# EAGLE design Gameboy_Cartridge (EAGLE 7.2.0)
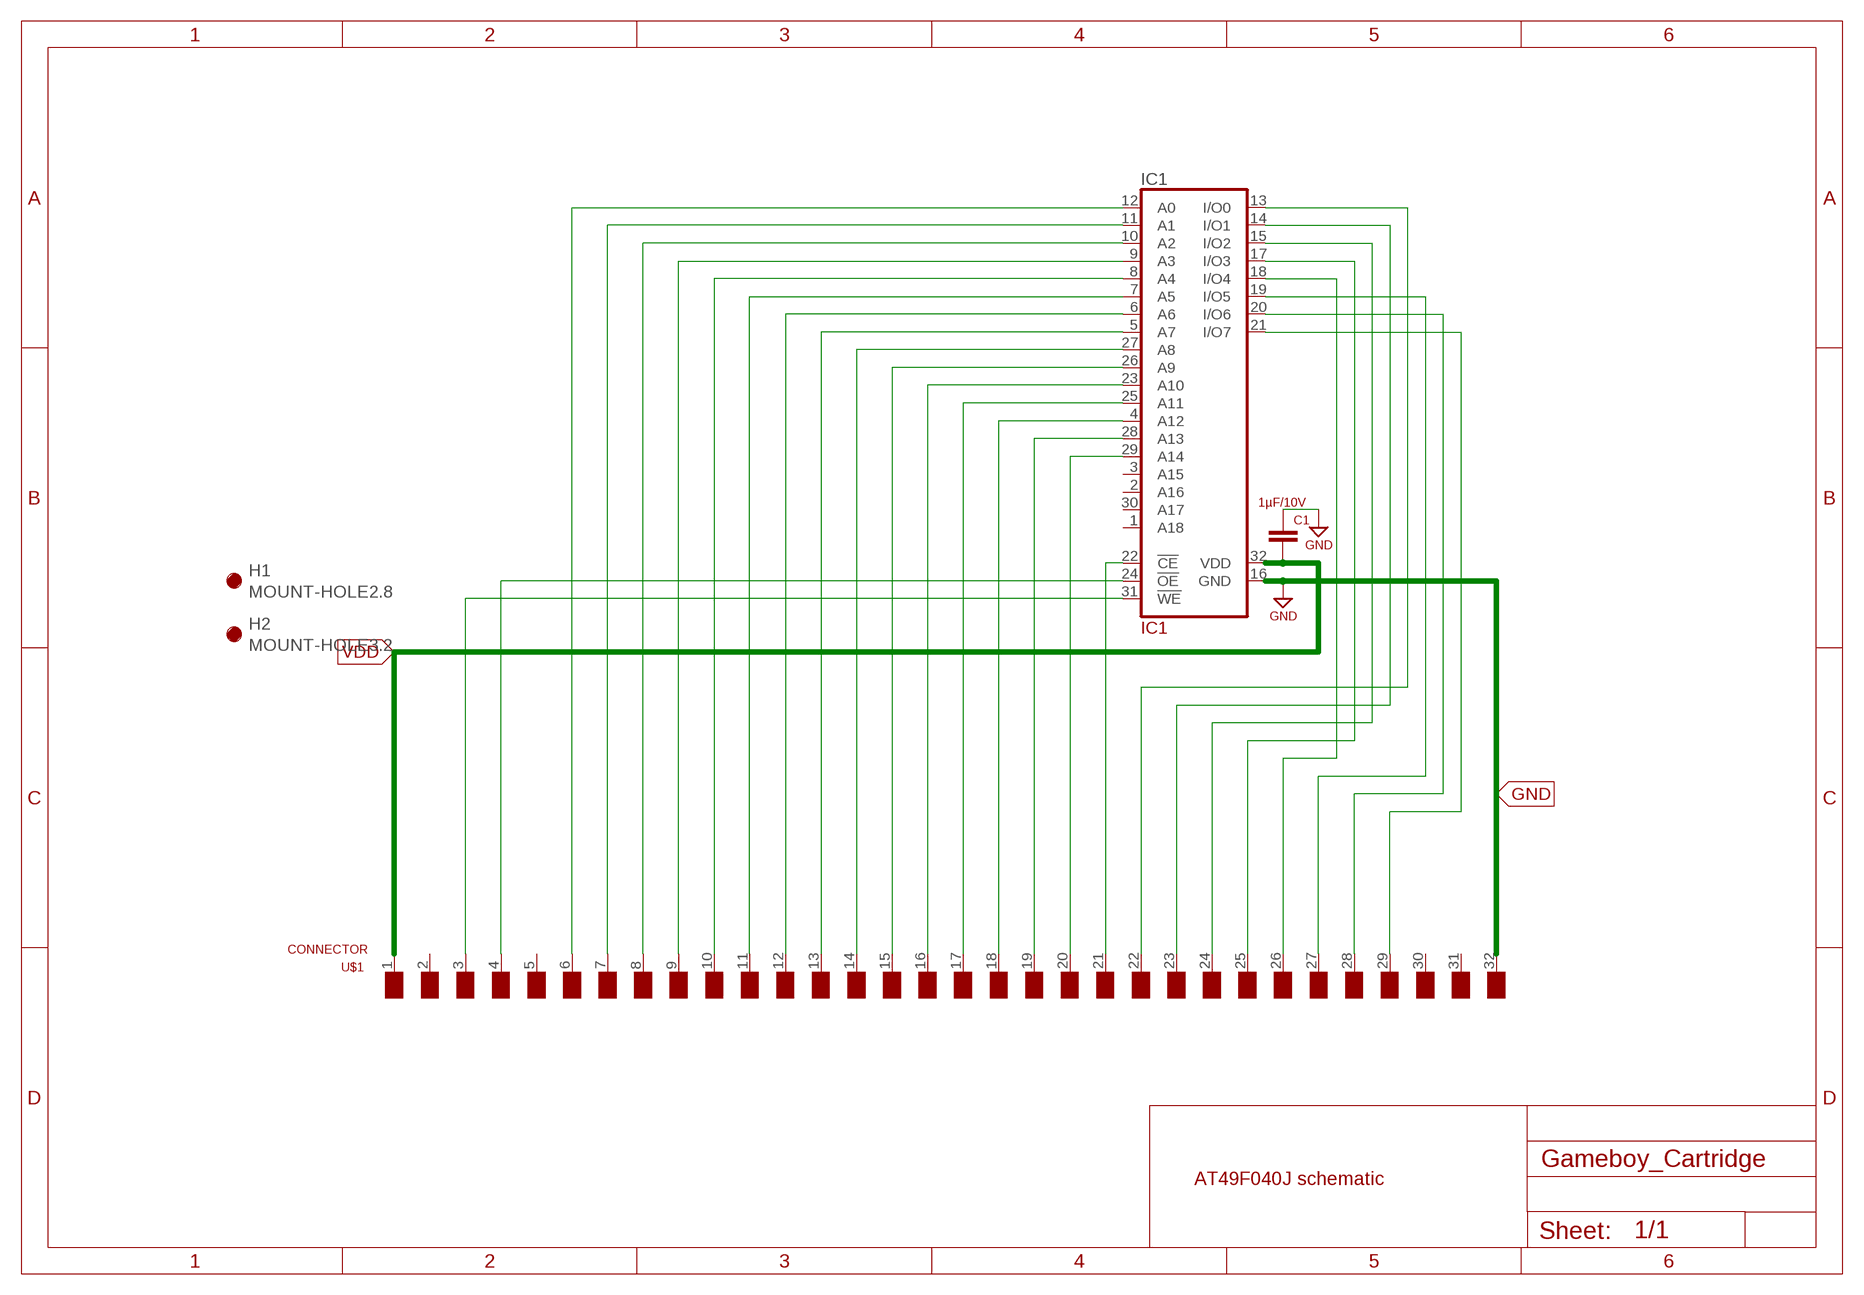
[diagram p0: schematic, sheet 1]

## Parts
C1  1µF/10V  C-EUC0603  [C0603]
H1  MOUNT-HOLE2.8  [2,8]
H2  MOUNT-HOLE3.2  [3,2]
IC1  IC1  AT49F040J  [PLCC32R]
U$1  CONNECTOR  [CONNECTOR]

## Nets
3: IC1.31(!WE) U$1.3(/WR)
4: IC1.24(!OE) U$1.4(/RD)
6: IC1.12(A0) U$1.6(A0)
7: IC1.11(A1) U$1.7(A1)
8: IC1.10(A2) U$1.8(A2)
9: IC1.9(A3) U$1.9(A3)
10: IC1.8(A4) U$1.10(A4)
11: IC1.7(A5) U$1.11(A5)
12: IC1.6(A6) U$1.12(A6)
13: IC1.5(A7) U$1.13(A7)
14: IC1.27(A8) U$1.14(A8)
15: IC1.26(A9) U$1.15(A9)
16: IC1.23(A10) U$1.16(A10)
17: IC1.25(A11) U$1.17(A11)
18: IC1.4(A12) U$1.18(A12)
19: IC1.28(A13) U$1.19(A13)
20: IC1.29(A14) U$1.20(A14)
21: IC1.22(!CE) U$1.21(A15)
22: IC1.13(I/O0) U$1.22(D0)
23: IC1.14(I/O1) U$1.23(D1)
24: IC1.15(I/O2) U$1.24(D2)
25: IC1.17(I/O3) U$1.25(D3)
26: IC1.18(I/O4) U$1.26(D4)
27: IC1.19(I/O5) U$1.27(D5)
28: IC1.20(I/O6) U$1.28(D6)
29: IC1.21(I/O7) U$1.29(D7)
GND: C1.1 IC1.16(GND) U$1.32(GND)
VDD: C1.2 IC1.32(VDD) U$1.1(VDD)
Unconnected: IC1.1(A18) IC1.2(A16) IC1.3(A15) IC1.30(A17) U$1.2(NC) U$1.5(/RCS) U$1.30(/RS) U$1.31(VIN)

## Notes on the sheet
- AT49F040J schematic

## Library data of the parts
C1 = resistor:C-EU: CAPACITOR, European symbol
H1 H2 = holes:MOUNT-HOLE: MOUNTING HOLE with drill center marker
IC1 = gameboy:AT49F040J: 4-Megabit FLASH MEMORY (512 K x 8 bit) 5 V-only
U$1 = gameboy:CONNECTOR: Connector Pads for Gameboy Cartridges

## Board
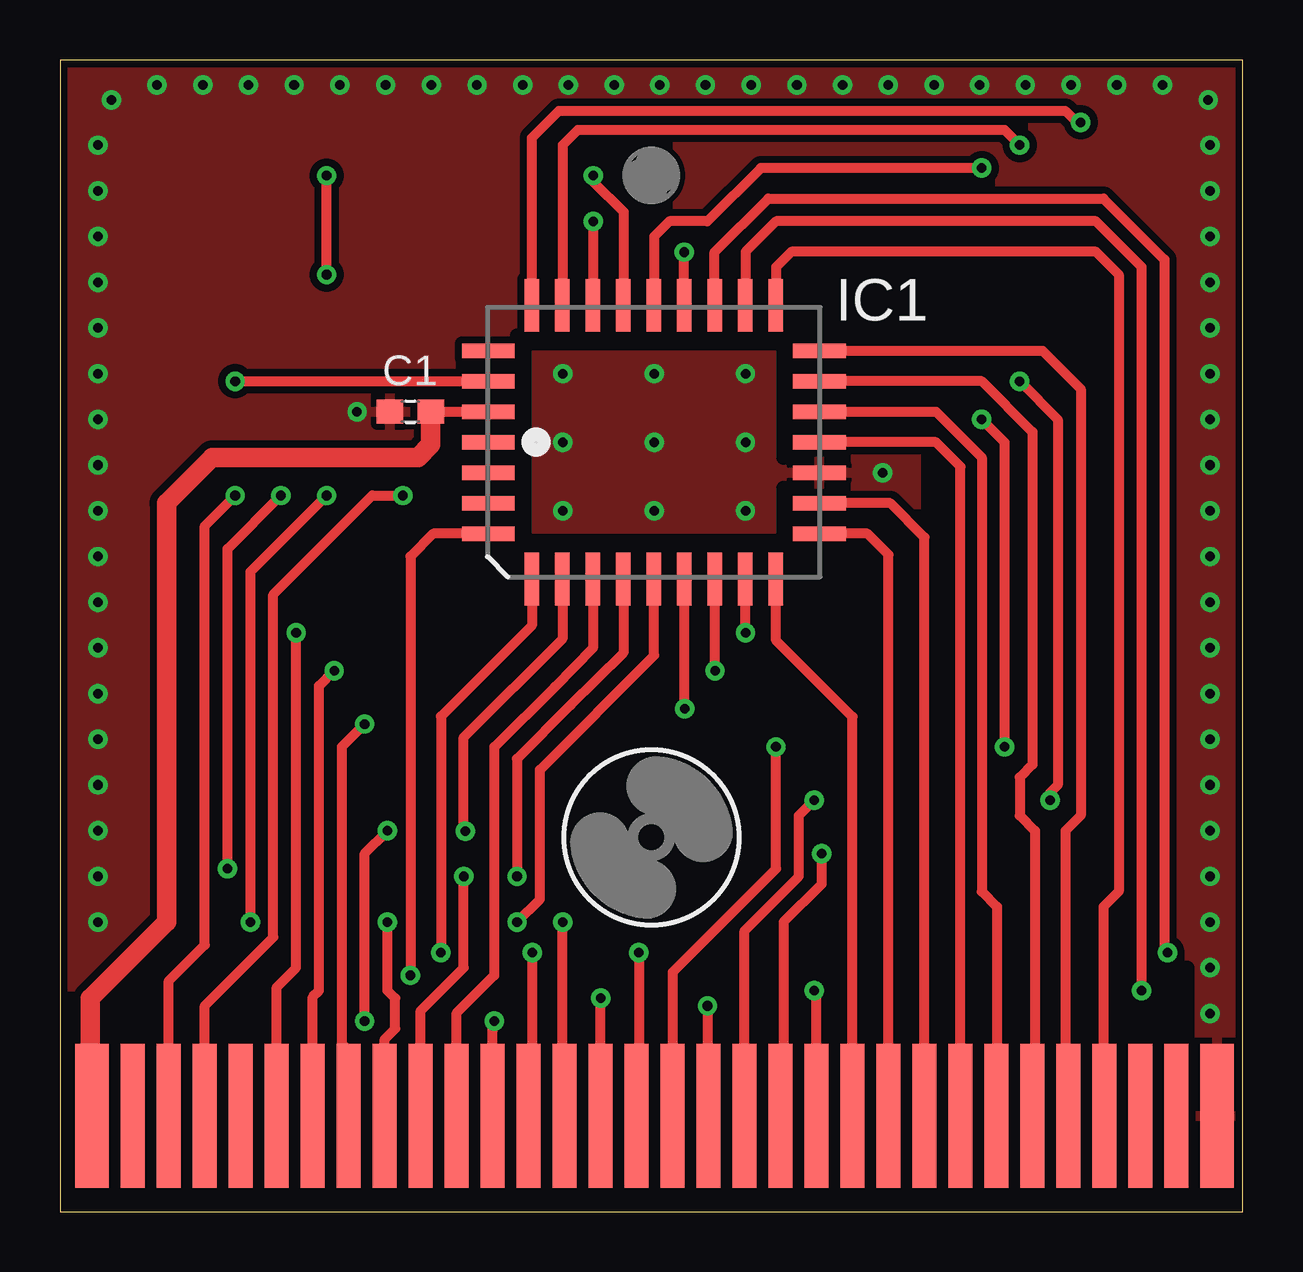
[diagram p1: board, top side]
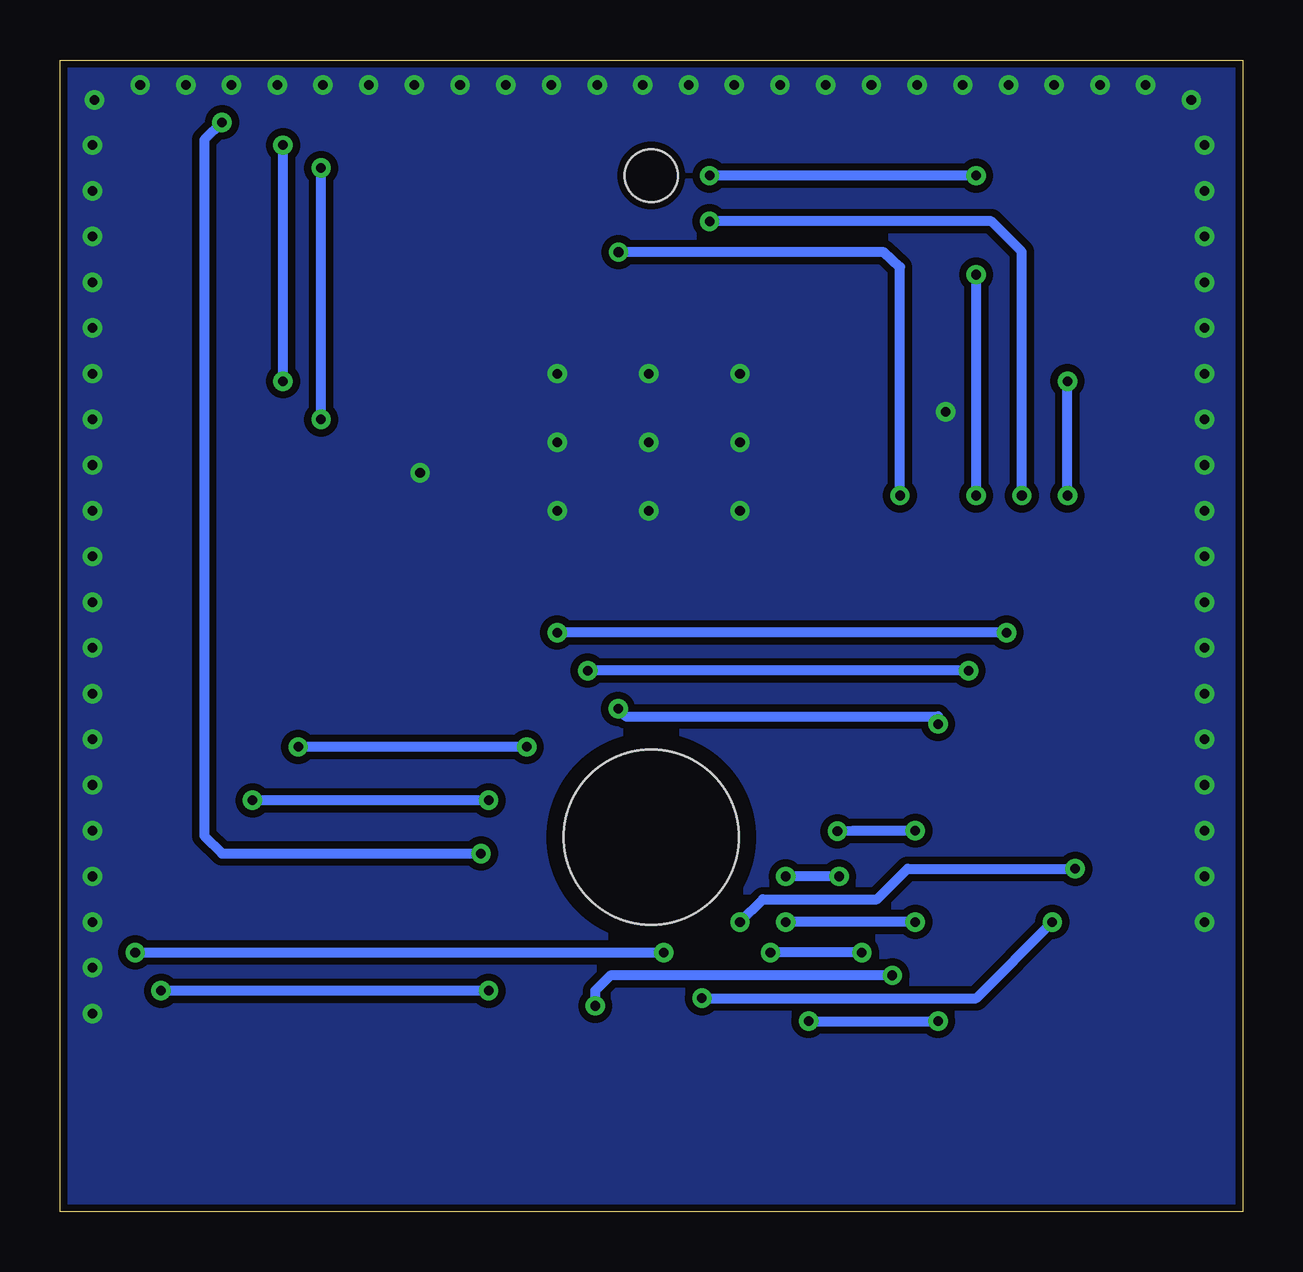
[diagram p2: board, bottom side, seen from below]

Size 49.3 x 48 mm. Coordinates in mm from the lower left corner, seen from the top.
Outline: 0,0 49.3,0 49.3,48 0,48 0,0
Copper layers (1*16): Top 0.035mm / dielectric 0.73mm / Bottom 0.035mm
Design rules "default *": minimum track width 10mil, minimum drill 15mil, track to track 8mil, track to pad 8mil, pad to pad 8mil, via to via 8mil, smd to smd 4mil, copper to edge 10mil, drill to drill 8mil, minimum pad ring 10mil, minimum via ring 8mil, stop-mask expansion 4mil, vias tented up to drill 0mil, thermal gap 10mil
tRestrict: area 36.2,7.3 to 37.1,31.4; area 43.8,7.3 to 44.8,13; area 44.8,7 to 47,10.2; area 19.1,27.6 to 19.4,36.5; area 19.1,36.2 to 30.5,36.5; area 19,27.6 to 30.8,27.9; area 30.2,31.4 to 30.5,36.2; area 30.2,27.6 to 30.5,30.2; area 47,0.3 to 48.9,1

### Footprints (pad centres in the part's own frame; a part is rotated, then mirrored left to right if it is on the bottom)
C0603 = smd 1.1 x 1: 1 -0.85,0; 2 0.85,0
2,8 = hole 2.2: 0,0
3,2 = hole 7.3: 0,0
PLCC32R = smd 0.6 x 2.2: 1 0,6.9; 2 -1.27,6.9; 3 -2.54,6.9; 4 -3.81,6.9; 14 -3.81,-6.9; 15 -2.54,-6.9; 16 -1.27,-6.9; 17 0,-6.9; 18 1.27,-6.9; 19 2.54,-6.9; 20 3.81,-6.9; 30 3.81,6.9; 31 2.54,6.9; 32 1.27,6.9 | smd 2.2 x 0.6: 5 -5.7,5.08; 6 -5.7,3.81; 7 -5.7,2.54; 8 -5.7,1.27; 9 -5.7,0; 10 -5.7,-1.27; 11 -5.7,-2.54; 12 -5.7,-3.81; 13 -5.7,-5.08; 21 5.7,-5.08; 22 5.7,-3.81; 23 5.7,-2.54; 24 5.7,-1.27; 25 5.7,0; 26 5.7,1.27; 27 5.7,2.54; 28 5.7,3.81; 29 5.7,5.08
CONNECTOR = smd 1.4 x 6: 1 0.7,-3; 32 47.6,-3 | smd 1 x 6: 2 2.4,-3; 3 3.9,-3; 4 5.4,-3; 5 6.9,-3; 6 8.4,-3; 7 9.9,-3; 8 11.4,-3; 9 12.9,-3; 10 14.4,-3; 11 15.9,-3; 12 17.4,-3; 13 18.9,-3; 14 20.4,-3; 15 21.9,-3; 16 23.4,-3; 17 24.9,-3; 18 26.4,-3; 19 27.9,-3; 20 29.4,-3; 21 30.9,-3; 22 32.4,-3; 23 33.9,-3; 24 35.4,-3; 25 36.9,-3; 26 38.4,-3; 27 39.9,-3; 28 41.4,-3; 29 42.9,-3; 30 44.4,-3; 31 45.9,-3

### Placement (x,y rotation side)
C1  14.61,33.34 0 top
H1  24.65,43.18 0 top
H2  24.65,15.6 0 top
IC1  24.75,32.07 90 top
U$1  0.64,6.99 0 top

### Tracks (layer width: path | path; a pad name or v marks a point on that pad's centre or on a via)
3  (via drill 0.4 pad 0.41)
  Top 0.406: U$1.3 4.54,9.62 6.03,11.11 6.03,28.57 v7.3,29.84 | v7.3,34.61 IC1.31
  Bottom 0.406: v7.3,29.84 v7.3,34.61
4  (via drill 0.4 pad 0.41)
  Top 0.406: U$1.4 6.04,8.57 8.89,11.43 8.89,25.72 13.02,29.84 v14.29,29.84 | 26.04,37.78 IC1.24 v26.02,39.99
  Bottom 0.406: v14.29,29.84 14.29,39.37 14.95,39.98 v26.02,39.99
6  (via drill 0.4 pad 0.41)
  Top 0.406: U$1.6 9.04,9.35 9.84,10.16 v9.84,24.13 | v28.57,24.13 28.57,26.35 IC1.12
  Bottom 0.406: v9.84,24.13 v28.57,24.13
7  (via drill 0.4 pad 0.41)
  Top 0.406: U$1.7 10.54,8.95 10.79,9.21 10.79,21.91 v11.43,22.54 | v27.3,22.54 27.3,26.35 IC1.11
  Bottom 0.406: v11.43,22.54 v27.3,22.54
8  (via drill 0.4 pad 0.41)
  Top 0.406: v26.04,20.95 26.04,26.35 IC1.10 | v12.7,20.32 11.75,19.37 11.75,6.99 12.06,6.67 12.06,4.01 U$1.8
  Bottom 0.406: v26.04,20.95 25.72,20.64 12.7,20.64 v12.7,20.32
9  (via drill 0.4 pad 0.41)
  Top 0.406: 13.54,11.95 v13.65,12.06 13.65,9.21 13.97,8.89 13.97,7.62 13.54,7.18 U$1.9 | v19.05,12.06 20,13.02 20,18.41 24.77,23.18 24.77,26.35 IC1.9
  Bottom 0.406: v13.65,12.06 v19.05,12.06
10  (via drill 0.4 pad 0.41)
  Top 0.406: IC1.8 23.48,23.28 21.29,21.11 19.05,18.87 v19.05,13.97 | U$1.10 15.04,8.37 16.83,10.16 v16.83,13.97
  Bottom 0.406: v16.83,13.97 v19.05,13.97
11
  Top 0.406: IC1.7 22.21,23.48 20.62,21.88 18.12,19.37 18.1,19.37 18.1,9.84 16.54,8.28 U$1.11
12  (via drill 0.4 pad 0.41)
  Top 0.406: IC1.6 20.94,23.88 16.83,19.76 16.83,15.88 16.8,15.85 v16.89,15.85 | U$1.12 18.04,7.56 v18.1,7.94 | v12.7,7.94 12.7,14.92 v13.65,15.88
  Bottom 0.406: v18.1,7.94 v12.7,7.94 | v13.65,15.88 16.23,15.88 v16.89,15.85
13  (via drill 0.4 pad 0.41)
  Top 0.406: v19.68,10.79 19.68,4.13 U$1.13 | IC1.5 19.67,24.43 15.88,20.64 v15.88,10.79
  Bottom 0.406: v15.88,10.79 v19.68,10.79
14  (via drill 0.4 pad 0.41)
  Top 0.406: v6.99,14.29 6.99,27.62 v9.21,29.84 | v22.23,41.27 22.23,37.78 IC1.27 | U$1.14 20.95,4.07 v20.95,12.06
  Bottom 0.406: v6.99,14.29 13.97,14.29 15.24,13.02 20,13.02 v20.95,12.06 | v9.21,29.84 9.21,40.01 10.48,41.27 v22.23,41.27
15  (via drill 0.4 pad 0.41)
  Top 0.406: U$1.15 22.54,8.58 v22.54,8.89 | v7.94,12.06 7.94,26.67 v11.11,29.84 | v11.11,39.05 v11.11,43.18 | v22.23,43.18 22.23,42.93 23.49,41.67 IC1.26
  Bottom 0.406: v22.54,8.89 11.11,8.89 v7.94,12.06 | v11.11,29.84 v11.11,39.05 | v11.11,43.18 v22.23,43.18
16  (via drill 0.4 pad 0.41)
  Top 0.406: IC1.23 27.29,39.99 29.53,42.23 43.5,42.23 46.04,39.69 46.04,10.92 v46.16,10.79 | v24.13,10.79 24.13,4.08 U$1.16
  Bottom 0.406: v46.16,10.79 v24.13,10.79
17  (via drill 0.4 pad 0.41)
  Top 0.406: v29.84,19.37 29.84,14.29 25.54,9.98 U$1.17 | v38.42,43.5 29.21,43.5 26.99,41.27 25.4,41.27 24.77,40.64 24.77,37.78 IC1.25 | v39.37,19.37 39.37,32.07 v38.42,33.02
  Bottom 0.406: v29.84,19.37 v39.37,19.37 | v38.42,33.02 v38.42,43.5
18  (via drill 0.4 pad 0.41)
  Top 0.406: IC1.4 15.56,28.26 14.61,27.3 v14.61,9.84 | v26.99,8.57 26.99,4.03 U$1.18
  Bottom 0.406: v14.61,9.84 26.35,9.84 26.99,9.21 v26.99,8.57
19  (via drill 0.4 pad 0.41)
  Top 0.406: U$1.19 28.54,11.71 30.8,13.97 30.8,16.51 v31.43,17.14 | IC1.28 20.95,37.78 20.95,44.45 21.59,45.09 39.37,45.09 v40.01,44.45 | v40.01,34.61 41.59,33.02 41.59,17.78 41.27,17.46 v41.27,17.14
  Bottom 0.406: v31.43,17.14 v41.27,17.14 | v40.01,34.61 v40.01,44.45
20  (via drill 0.4 pad 0.41)
  Top 0.406: IC1.29 19.67,44.75 20.8,45.88 41.9,45.88 42.38,45.4 v42.55,45.4 | U$1.20 30.16,4.11 30.16,12.06 31.75,13.65 v31.75,14.92
  Bottom 0.406: v31.75,14.92 42.55,14.92 43.28,15.66 43.28,44.67 v42.55,45.4
21  (via drill 0.4 pad 0.41)
  Top 0.406: U$1.21 31.54,9.11 v31.43,9.21 | v45.09,9.21 45.09,39.37 43.18,41.27 29.84,41.27 28.57,40.01 28.57,37.78 IC1.22
  Bottom 0.406: v31.43,9.21 v45.09,9.21
22
  Top 0.406: U$1.22 33.03,20.62 29.84,23.81 29.84,26.35 IC1.13
23
  Top 0.406: U$1.23 34.53,27.38 33.66,28.26 IC1.14
24
  Top 0.406: U$1.24 36.03,28.1 34.61,29.53 IC1.15
25
  Top 0.406: U$1.25 37.53,31.05 36.51,32.07 IC1.17
26
  Top 0.406: IC1.18 36.51,33.34 38.42,31.43 38.42,13.34 39.05,12.7 39.05,4 U$1.26
27
  Top 0.406: IC1.19 38.42,34.61 40.53,32.49 40.53,18.63 40.01,18.1 40.01,16.51 40.64,15.88 40.64,4.09 U$1.27
28
  Top 0.406: U$1.28 41.91,4.11 41.91,15.88 42.55,16.51 42.55,34.29 40.96,35.88 IC1.20
29
  Top 0.406: IC1.21 29.84,37.78 29.84,39.37 30.48,40.01 43.18,40.01 44.13,39.05 44.13,13.34 43.5,12.7 43.5,4.02 U$1.29
GND  (via drill 0.4)
  other vias: 2.14,46.33 4.05,46.97 5.95,46.97 7.86,46.97 9.76,46.97 11.67,46.97 13.57,46.97 15.48,46.97 17.38,46.97 19.29,46.97 21.19,46.97 23.1,46.97 25,46.97 28.81,46.97 30.72,46.97 32.62,46.97 34.53,46.97 36.43,46.97 38.34,46.97 40.24,46.97 42.15,46.97 44.05,46.97 45.96,46.97 47.94,33.02 47.94,31.11 47.94,29.21 47.94,27.3 47.94,25.4 47.94,23.5 47.94,21.59 47.94,19.68 47.94,17.78 47.94,15.88 47.94,13.97 47.94,12.06 47.94,10.16 47.94,8.26 1.59,33.02 1.59,31.11 1.59,29.21 1.59,27.3 1.59,25.4 1.59,23.5 1.59,21.59 1.59,19.68 1.59,17.78 1.59,15.88 1.59,13.97 1.59,12.06 20.95,34.92 24.77,34.92 28.57,34.92 28.57,32.07 28.57,29.21 24.77,29.21 20.95,29.21 20.95,32.07 24.77,32.07 26.91,46.97 1.59,34.92 1.59,36.83 47.94,36.83 47.94,34.92 47.86,46.33 1.59,38.73 1.59,40.64 1.59,42.55 1.59,44.45 47.94,38.73 47.94,40.64 47.94,42.55 47.94,44.45 34.29,30.8 12.38,33.34
  pour Top (isolate 0.305): 0,49.53 49.53,49.53 49.53,0 0,0
  pour Bottom (isolate 0.305): 0,49.53 49.53,49.53 49.53,0 0,0
VDD
  Top 0.406: C1.2 IC1.32 | 1.27,4.05 U$1.1
  Top 0.813: C1.2 15.46,31.96 14.92,31.43 6.35,31.43 4.45,29.53 4.45,12.06 1.27,8.89 1.27,4.05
